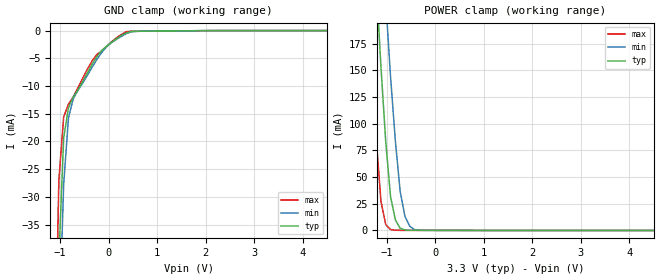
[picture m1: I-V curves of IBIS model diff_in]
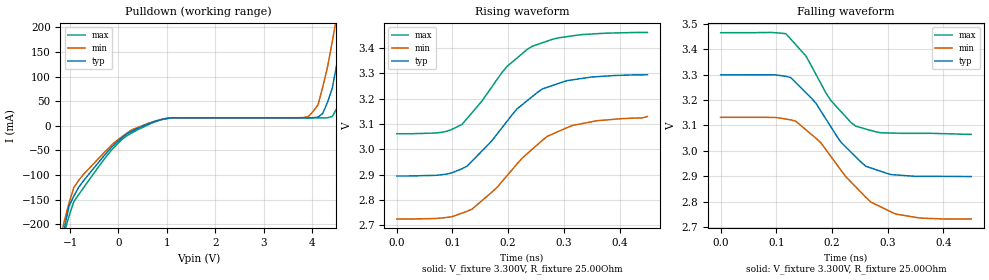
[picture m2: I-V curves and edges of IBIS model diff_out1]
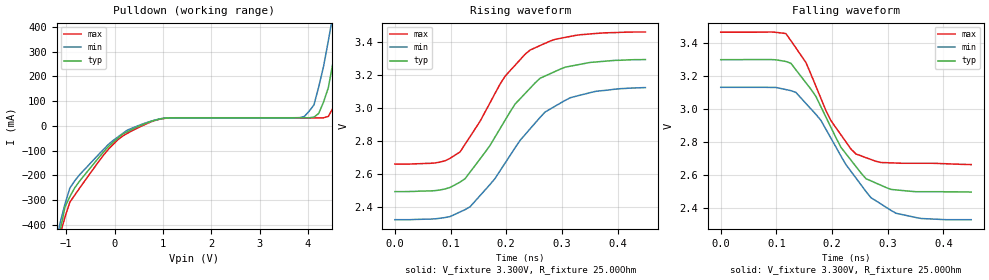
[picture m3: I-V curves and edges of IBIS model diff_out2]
|   National Semiconductor Corporation
|   IBIS Model of DS15BA101
[IBIS Ver]   3.2
[Comment char]  |_char
[File name]   ds15ba101.ibs
[File Rev]   1.1
[Date]   1/26/2009
[Source]   From silicon level SPICE model
[Notes]
|   This IBIS model uses the Model Selector keyword to allow
|   selection of the 400 mV or 800 mV output for the OUT pins.
|   Most EDA tools will automatically allow you to select which
|   model to use.
[Disclaimer]
(C) Copyright National Semiconductor Corporation 2008
   All rights reserved
   National Semiconductor Corporation hereby grants
the user of this IBIS model a non-exclusive, nontransferable
license to use this IBIS model under the following terms.
Before using this IBIS model, the user should read this
license.  If the user does not accept these terms,  the
IBIS model should be returned to National within 30 days.
   The user is granted this license only to use the
IBIS model and is not granted rights to sell, load, rent,
lease or license the IBIS model in whole or in part, or in
modified form to anyone other than user. User may modify
the IBIS model to suit its specific applications but rights
to derivative works and such modifications shall belong to
National.
   This IBIS model is provided on an "AS IS" basis and
National makes absolutely no warranty with respect to the
information contained herein.NATIONAL DISCLAIMS AND CUSTOMER
WAIVES ALL WARRANTIES, EXPRESS OR IMPLIED, INCLUDING
WARRANTIES OF MERCHANTABILITY OR FITNESS FOR A PARTICULAR
PURPOSE. The entire risk as to quality and performance is
with the Customer. ACCORDINGLY, IN NO EVENT SHALL THE
COMPANY BE LIABLE FOR ANY DAMAGES, WHETHER IN CONTRACT OR
TORT,INCLUDING ANY LOST PROFITS OR OTHER INCIDENTAL,
CONSEQUENTIAL, EXEMPLARY, OR PUNITIVE DAMAGES ARISING OUT
OF THE USE OR APPLICATION OF THE IBIS model provided in
this package.Further, National reserves the right to make
changes without notice to any product herein to improve
reliability, function, or design. National does not convey
any license under patent rights or any other intellectual
property rights, including those of third parties.
   National is not obligated to provide maintenance or support
for the licensed IBIS model.
Contact National at ATTN:INTERFACE APPLICATIONS/IBIS MODELS.
2900 Semiconductor Drive, M/S E-170, Santa Clara, CA 95052-8090
[Component]   DS15BA101
[Manufacturer]  National Semiconductor
[Package]
|   typ   min   max
R_pkg   388e-3   388e-3   388e-3
L_pkg   8.890e-10   8.890e-10   8.890e-10
C_pkg   2.575e-13   2.575e-13   2.575e-13
[PIN]   signal_name   model_name   R_pin   L_pin   C_pin
1   IN+   diff_in   0.376   8.66e-10   2.49e-13
2   IN-   diff_in   0.380   8.66e-10   2.62e-13
3   Vee   GND
4   Rvo   NC
5   Vcc   POWER
6   Vee   GND
7   OUT-   out_select   0.402   9.05e-10   2.66e-13
8   OUT+   out_select   0.394   9.20e-10   2.53e-13
DAP   Vee   GND
[Diff_pin]   inv_pin   vdiff   tdelay_typ   tdelay_min   tdelay_max
| The '+' pin is Diff_pin and the '-' pin is the inv_pin
1   2   0.050   0 0 0
8   7   0.000   0 0 0
[Model Selector] out_select
diff_out1 OUT with 400mV amplitude (Rvo = 953 ohms)
diff_out2 OUT with 800mV amplitude (Rvo = 487 ohms)
| Models and submodels in the file (3): diff_in (Input), diff_out1 (Open_sink), diff_out2 (Open_sink)
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[Model]   diff_in
Model_type   Input
| Differential input thresholds under [Diff_pin] over rides Vinl/Vinh
Vinl=0.8V
Vinh=2.0V
|   typ   min   max
C_comp   2.100pF   2.000pF   2.200pF
[Voltage Range]   3.300V   3.135   3.465
[Temperature Range]   25.0   85.0   -40.0
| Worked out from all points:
|   POWER clamp passes 1 mA (typ) near -0.66 V on its own axis
[GND Clamp]
|Voltage   I(typ)   I(min)   I(max)
-3.399V   -2.254A    -2.073A    -2.497A
-1.122V   -87.32mA   -103.5mA   -68.63mA
-1.023V   -41mA      -55.58mA   -26.98mA
-924mV    -19.37mA   -27.73mA   -15.57mA
-825mV    -13.9mA    -15.75mA   -13.27mA
-726mV    -11.99mA   -12.29mA   -11.95mA
-429mV    -7.509mA   -7.972mA   -6.844mA
-231mV    -4.591mA   -5.09mA    -4.239mA
-33mV     -2.779mA   -2.858mA   -2.793mA
363mV     -421.5uA   -558.8uA   -206.1uA
1.947V    -14.7uA    -3.4uA     -21.9uA
6.798V    0A         0A         0A
[Power Clamp]
|Voltage   I(typ)   I(min)   I(max)
-3.399V   2.394A     2.359A     2.462A
-1.419V   411.2mA    540.1mA    263.8mA
-1.32V    320.6mA    455.3mA    169.6mA
-1.221V   234.4mA    371.9mA    86.99mA
-1.122V   153.4mA    291.2mA    27.36mA
-1.023V   83.04mA    214.7mA    5.505mA
-924mV    31.7mA     144mA      863.7uA
-825mV    10.07mA    83.98mA    275.9uA
-726mV    2.047mA    36.65mA    133.4uA
-627mV    479.1uA    13.13mA    126.4uA
-429mV    139.2uA    763.4uA    115uA
6.798V    0A         0A         0A
[Model]   diff_out1
Model_type   Open_sink
Vmeas = 3.1V   | Single-Ended Crossing Point for OUT+ and OUT-
Vref = 3.3V
Cref = 0.000F
Rref = 25.000Ohm
|   typ   min   max
C_comp   0.800pF   0.700pF   1.300pF
[Voltage Range]   3.300V   3.135   3.465
[Temperature Range]   25.0   85.0   -40.0
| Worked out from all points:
|   slope of the pulldown table from 0 to 0.495 V, typ, clamps not added: 16.8 ohm
|   falling waveform, V_fixture 3.300V, R_fixture 25.00Ohm: 20-80 % time 83.8ps typ, 93.3ps min, 71.8ps max; typ from 3.3 V to 2.9 V
|   rising waveform, V_fixture 3.300V, R_fixture 25.00Ohm: 20-80 % time 102ps typ, 111ps min, 93.2ps max; typ from 2.9 V to 3.29 V
[Pulldown]
|Voltage   I(typ)   I(min)   I(max)
-3.399V   -1.929A    -1.747A    -2.18A
-1.122V   -210mA     -194.4mA   -217.8mA
-825mV    -125.4mA   -111.2mA   -140.1mA
165mV     -16.77mA   -15.63mA   -20.85mA
1.056V    15.74mA    15.69mA    15.31mA
3.927V    16.29mA    18.94mA    15.99mA
4.125V    17.41mA    42.22mA    15.99mA
4.422V    76.83mA    171.3mA    18.91mA
4.521V    128.9mA    226.1mA    36.48mA
4.62V     184.3mA    284.4mA    82.16mA
4.818V    312.6mA    405.5mA    207.2mA
6.798V    1.746A     1.72A      1.795A
[Ramp]
R_load = 25.00Ohm
|   typ   min   max
dV/dt_r   0.38/100p   0.38/100p   0.38/100p
dV/dt_f   0.38/100p   0.38/100p   0.38/100p
[Falling Waveform]
V_fixture = 3.300V
V_fixture_min = 3.135V
V_fixture_max = 3.465V
R_fixture = 25.00Ohm
|Time   V(typ)   V(min)   V(max)
0s        3.299V     3.132V     3.465V
117ps     3.294V     3.125V     3.461V
135ps     3.268V     3.117V     3.418V
153ps     3.229V     3.083V     3.374V
180ps     3.157V     3.032V     3.265V
216ps     3.034V     2.924V     3.155V
243ps     2.976V     2.858V     3.097V
270ps     2.933V     2.798V     3.08V
315ps     2.905V     2.751V     3.07V
450ps     2.899V     2.732V     3.065V
[Rising Waveform]
V_fixture = 3.300V
V_fixture_min = 3.135V
V_fixture_max = 3.465V
R_fixture = 25.00Ohm
|Time   V(typ)   V(min)   V(max)
0s        2.895V     2.725V     3.062V
81ps      2.9V       2.729V     3.068V
117ps     2.924V     2.748V     3.098V
135ps     2.954V     2.764V     3.145V
198ps     3.111V     2.896V     3.328V
216ps     3.16V      2.943V     3.361V
243ps     3.208V     3V         3.407V
270ps     3.245V     3.051V     3.428V
315ps     3.275V     3.094V     3.448V
450ps     3.295V     3.13V      3.462V
[Model]   diff_out2
Model_type   Open_sink
Vmeas = 3.1V   | Single-Ended Crossing Point for OUT+ and OUT-
Vref = 3.3V
Cref = 0.000F
Rref = 25.000Ohm
|   typ   min   max
C_comp   0.800pF   0.700pF   1.300pF
[Voltage Range]   3.300V   3.135   3.465
[Temperature Range]   25.0   85.0   -40.0
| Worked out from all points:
|   slope of the pulldown table from 0 to 0.495 V, typ, clamps not added: 8.38 ohm
|   falling waveform, V_fixture 3.300V, R_fixture 25.00Ohm: 20-80 % time 83.8ps typ, 93.3ps min, 71.8ps max; typ from 3.3 V to 2.5 V
|   rising waveform, V_fixture 3.300V, R_fixture 25.00Ohm: 20-80 % time 102ps typ, 110ps min, 93.2ps max; typ from 2.5 V to 3.29 V
[Pulldown]
|Voltage   I(typ)   I(min)   I(max)
-3.399V   -3.858A    -3.495A    -4.36A
-1.122V   -420.1mA   -388.9mA   -435.5mA
-825mV    -250.8mA   -222.4mA   -280.1mA
165mV     -33.53mA   -31.27mA   -41.7mA
1.056V    31.47mA    31.37mA    30.62mA
3.927V    32.57mA    37.89mA    31.97mA
4.125V    34.82mA    84.44mA    31.97mA
4.422V    153.7mA    342.7mA    37.81mA
4.521V    257.7mA    452.3mA    72.95mA
4.62V     368.6mA    568.9mA    164.3mA
4.818V    625.2mA    811mA      414.4mA
6.798V    3.491A     3.44A      3.591A
[Ramp]
R_load = 25.00Ohm
|   typ   min   max
dV/dt_r   0.38/100p   0.38/100p   0.38/100p
dV/dt_f   0.38/100p   0.38/100p   0.38/100p
[Falling Waveform]
V_fixture = 3.300V
V_fixture_min = 3.135V
V_fixture_max = 3.465V
R_fixture = 25.00Ohm
|Time   V(typ)   V(min)   V(max)
0s        3.299V     3.132V     3.465V
117ps     3.288V     3.118V     3.457V
135ps     3.238V     3.101V     3.37V
153ps     3.16V      3.035V     3.282V
180ps     3.014V     2.932V     3.065V
216ps     2.769V     2.716V     2.845V
243ps     2.653V     2.584V     2.729V
270ps     2.567V     2.465V     2.696V
315ps     2.512V     2.371V     2.674V
450ps     2.499V     2.332V     2.665V
[Rising Waveform]
V_fixture = 3.300V
V_fixture_min = 3.135V
V_fixture_max = 3.465V
R_fixture = 25.00Ohm
|Time   V(typ)   V(min)   V(max)
0s        2.495V     2.325V     2.662V
81ps      2.505V     2.334V     2.674V
117ps     2.553V     2.372V     2.735V
135ps     2.613V     2.403V     2.828V
198ps     2.928V     2.668V     3.194V
216ps     3.026V     2.761V     3.261V
243ps     3.121V     2.876V     3.353V
270ps     3.196V     2.978V     3.393V
315ps     3.255V     3.064V     3.435V
450ps     3.295V     3.125V     3.462V
